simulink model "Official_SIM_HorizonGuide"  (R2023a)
settings: Solver=ode4  StartTime=0.0  StopTime=100  FixedStep=0.01  RelTol=1e-3
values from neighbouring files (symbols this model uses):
  Aeq = zeros(6*N+3*(N-1),6*N+3*(N-1))    [Input_Official_SIM.m]
  c = 1e-4    (= 0.0001)    [Input_Official_SIM.m]
  dt = 8    [Input_Official_SIM.m]
  dyn_s = 1e3    (= 1000)    [Input_Official_SIM.m]
  F_D = -1/2*rho*CD*S*Vx^2    (= -0.0398770126883)    [Input_Official_SIM.m]
  Fj2 = -m_c*((3*J2*mu*(r_E^2))/(2*(r^4)))    (= -0.00135234249549)    [Input_Official_SIM.m]
  G = c*(lambda_low-lambda_top)/(sigma_0)    (= -0.03998)    [Input_Official_SIM.m]
  K_v = 20    [Input_Official_SIM.m]
  k_x = 2    [Input_Official_SIM.m]
  k_y = 0.2    [Input_Official_SIM.m]
  k_z = 2    [Input_Official_SIM.m]
  KF = 12.5*2    (= 25)    [Input_Official_SIM.m]
  lambda_low = 0.0001    [Input_Official_SIM.m]
  lambda_top = 0.2    [Input_Official_SIM.m]
  m_c = 130    [Input_Official_SIM.m]
  m_c0 = 130    [Input_Official_SIM.m]
  N = 20    [Input_Official_SIM.m]
  omega_0 = (mu/r^3)^0.5    (= 0.00105684438429)    [Input_Official_SIM.m]
  sigma_0 = 5e-4    (= 0.0005)    [Input_Official_SIM.m]
  tau = 1    [Input_Official_SIM.m]
  U_off = 0.2    [Input_Official_SIM.m]
  U_on = 0.75    [Input_Official_SIM.m]
  Umax = 2    [Input_Official_SIM.m]
  updaterate = 2    [Input_Official_SIM.m]
  x0 = -200    [Input_Official_SIM.m]
  x0_dot = 3/2*omega_0*z0    (= 0.158526657643)    [Input_Official_SIM.m]
  y0 = 0    [Input_Official_SIM.m]
  y0_dot = 0    [Input_Official_SIM.m]
  z0 = 100    [Input_Official_SIM.m]
  z0_dot = 0    [Input_Official_SIM.m]
undefined symbols (not defined in the file or in its folder): DiscIntNeverNeededParam

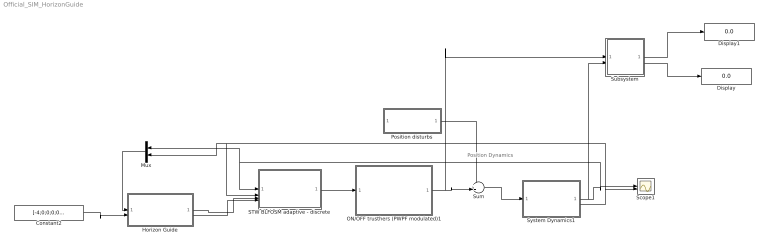
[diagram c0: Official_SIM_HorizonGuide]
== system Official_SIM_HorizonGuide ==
  note: Position Dynamics
  Constant2 : Constant  Value=[-4;0;0;0;0;0]
  Display : Display
  Display1 : Display
  Horizon Guide : Subsystem  TreatAsAtomicUnit=on
  Mux : Mux  Inputs=2
  ON/OFF trusthers (PWPF modulated)1 : Subsystem
  Position disturbs : Subsystem
  STW BLFOSM adaptive - discrete : Subsystem  TreatAsAtomicUnit=on  SystemSampleTime=0.1
  Scope1 : Scope  NumInputPorts=2
  Subsystem : Subsystem
  Sum : Sum  Inputs=++|
  System Dynamics1 : Subsystem
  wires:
  Horizon Guide/1(x_Des) -> STW BLFOSM adaptive - discrete/3(x_des)
  System Dynamics1/2(x_dot) -> STW BLFOSM adaptive - discrete/2(x_dot_live), Mux/2, Scope1/2
  Constant2/1 -> Horizon Guide/2(x_target)
  Sum/1 -> System Dynamics1/1(F)
  Mux/1 -> Horizon Guide/1(x_start)
  Horizon Guide/2(x_dot_dest) -> STW BLFOSM adaptive - discrete/4(x_dot_des)
  System Dynamics1/1(x) -> Subsystem/2(x), STW BLFOSM adaptive - discrete/1(x_live), Mux/1, Scope1/1
  Position disturbs/1(Out1) -> Sum/1
  STW BLFOSM adaptive - discrete/1(Trust) -> ON/OFF trusthers (PWPF modulated)1/1(In1)
  ON/OFF trusthers (PWPF modulated)1/1(F) -> Subsystem/1(F), Sum/2
  Subsystem/2(Endtime) -> Display/1
  Subsystem/1(Prop) -> Display1/1

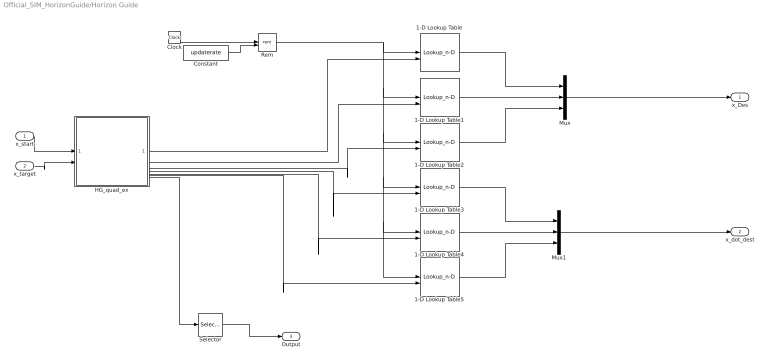
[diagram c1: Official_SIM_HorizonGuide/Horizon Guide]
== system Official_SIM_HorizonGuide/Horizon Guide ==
  x_start : Inport
  x_target : Inport  Port=2
  1-D Lookup Table{,1..5} (6 alike) : Lookup_n-D  NumberOfTableDimensions=1  BreakpointsForDimension1=[0:dt:(N-1)*dt]  TableSource=Input port  Table=tanh([-5:5])  InterpMethod=Cubic spline  InternalRulePriority=Speed  RndMeth=Simplest
  Clock : Clock
  Constant : Constant  Value=updaterate
  HG_quad_ex : MATLAB Function  TreatAsAtomicUnit=on  SystemSampleTime=updaterate
  Mux : Mux  Inputs=3
  Mux1 : Mux  Inputs=3
  Rem : Math  Operator=rem
  Selector : Selector  NumberOfDimensions=2  InputPortWidth=3  IndexOptions=Index vector (dialog),Index vector (dialog)  Indices=[1:3],1  OutputSizes=1,1
  x_Des : Outport
  x_dot_dest : Outport  Port=2
  Output : Outport  Port=3
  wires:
  Constant/1 -> Rem/2
  Rem/1 -> 1-D Lookup Table5/1, 1-D Lookup Table4/1, 1-D Lookup Table3/1, 1-D Lookup Table2/1, 1-D Lookup Table1/1, 1-D Lookup Table/1
  Clock/1 -> Rem/1
  Mux/1 -> x_Des/1
  Mux1/1 -> x_dot_dest/1
  1-D Lookup Table/1 -> Mux/1
  1-D Lookup Table1/1 -> Mux/2
  1-D Lookup Table2/1 -> Mux/3
  1-D Lookup Table3/1 -> Mux1/1
  1-D Lookup Table4/1 -> Mux1/2
  1-D Lookup Table5/1 -> Mux1/3
  HG_quad_ex/1(x) -> 1-D Lookup Table/2
  HG_quad_ex/2(y) -> 1-D Lookup Table1/2
  HG_quad_ex/3(z) -> 1-D Lookup Table2/2
  HG_quad_ex/4(x_dot) -> 1-D Lookup Table3/2
  HG_quad_ex/5(y_dot) -> 1-D Lookup Table4/2
  HG_quad_ex/6(z_dot) -> 1-D Lookup Table5/2
  HG_quad_ex/7(u) -> Selector/1
  Selector/1 -> Output/1
  x_start/1 -> HG_quad_ex/1(x_start)
  x_target/1 -> HG_quad_ex/2(x_target)

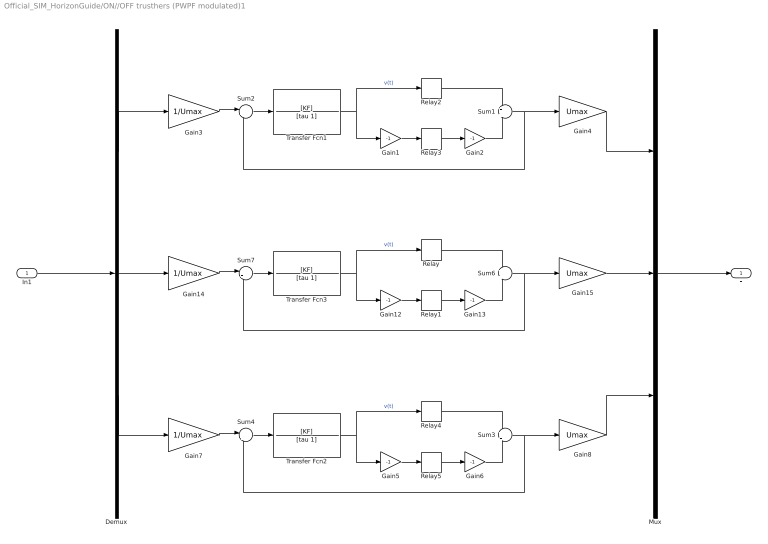
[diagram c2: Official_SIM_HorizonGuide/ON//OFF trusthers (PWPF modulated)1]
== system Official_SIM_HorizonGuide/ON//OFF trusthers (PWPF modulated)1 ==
  In1 : Inport
  Demux : Demux  Outputs=3
  Gain{1..2,5..6,12..13} (6 alike) : Gain  Gain=-1
  Gain14 : Gain  Gain=1/Umax  Multiplication=Matrix(K*u)
  Gain15 : Gain  Gain=Umax  Multiplication=Matrix(K*u)
  Gain3 : Gain  Gain=1/Umax  Multiplication=Matrix(K*u)
  Gain4 : Gain  Gain=Umax  Multiplication=Matrix(K*u)
  Gain7 : Gain  Gain=1/Umax  Multiplication=Matrix(K*u)
  Gain8 : Gain  Gain=Umax  Multiplication=Matrix(K*u)
  Mux : Mux  Inputs=3
  Relay{,1..5} (6 alike) : Relay  OnSwitchValue=U_on  OffSwitchValue=U_off
  Sum1 : Sum  Inputs=+|+
  Sum2 : Sum  Inputs=|+-
  Sum3 : Sum  Inputs=+|+
  Sum4 : Sum  Inputs=|+-
  Sum6 : Sum  Inputs=+|+
  Sum7 : Sum  Inputs=|+-
  Transfer Fcn1 : TransferFcn  Numerator=[KF]  Denominator=[tau 1]
  Transfer Fcn2 : TransferFcn  Numerator=[KF]  Denominator=[tau 1]
  Transfer Fcn3 : TransferFcn  Numerator=[KF]  Denominator=[tau 1]
  F : Outport
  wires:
  Relay/1 -> Sum6/1
  In1/1 -> Demux/1
  Relay3/1 -> Gain2/1
  Demux/3 -> Gain7/1
  Demux/2 -> Gain14/1
  Sum2/1 -> Transfer Fcn1/1
  Relay2/1 -> Sum1/1
  Sum7/1 -> Transfer Fcn3/1
  Gain6/1 -> Sum3/2
  Relay5/1 -> Gain6/1
  Gain2/1 -> Sum1/2
  Sum6/1 -> Gain15/1, Sum7/2
  Relay1/1 -> Gain13/1
  Sum3/1 -> Gain8/1, Sum4/2
  Gain7/1 -> Sum4/1
  Gain12/1 -> Relay1/1
  Transfer Fcn2/1 -> Gain5/1, Relay4/1  "v(t)"
  Gain1/1 -> Relay3/1
  Gain5/1 -> Relay5/1
  Sum1/1 -> Gain4/1, Sum2/2
  Gain13/1 -> Sum6/2
  Relay4/1 -> Sum3/1
  Sum4/1 -> Transfer Fcn2/1
  Transfer Fcn3/1 -> Gain12/1, Relay/1  "v(t)"
  Gain3/1 -> Sum2/1
  Transfer Fcn1/1 -> Gain1/1, Relay2/1  "v(t)"
  Gain14/1 -> Sum7/1
  Gain15/1 -> Mux/2
  Gain4/1 -> Mux/1
  Gain8/1 -> Mux/3
  Demux/1 -> Gain3/1
  Mux/1 -> F/1

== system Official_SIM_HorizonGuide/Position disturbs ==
  Constant : Constant  Value=F_D+Fj2
  Constant1 : Constant  Value=0
  Constant2 : Constant  Value=0
  Mux : Mux  Inputs=3
  Out1 : Outport
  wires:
  Constant/1 -> Mux/1
  Mux/1 -> Out1/1
  Constant1/1 -> Mux/2
  Constant2/1 -> Mux/3

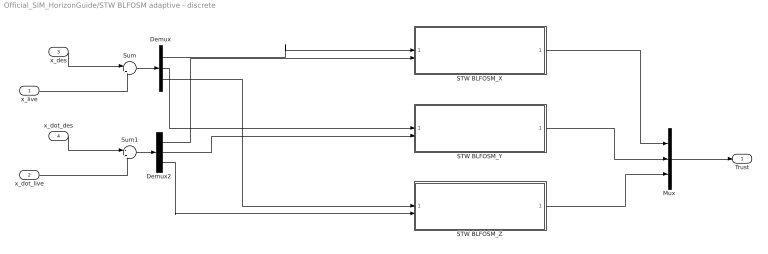
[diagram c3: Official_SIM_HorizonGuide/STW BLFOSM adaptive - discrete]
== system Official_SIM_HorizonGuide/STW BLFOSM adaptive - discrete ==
  x_live : Inport
  x_dot_live : Inport  Port=2
  x_des : Inport  Port=3
  x_dot_des : Inport  Port=4
  Demux : Demux  Outputs=3
  Demux2 : Demux  Outputs=3
  Mux : Mux  Inputs=3
  STW BLFOSM_X : Subsystem
  STW BLFOSM_Y : Subsystem
  STW BLFOSM_Z : Subsystem
  Sum : Sum  Inputs=-|+
  Sum1 : Sum  Inputs=-|+
  Trust : Outport
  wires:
  STW BLFOSM_Z/1(T_X) -> Mux/3
  STW BLFOSM_Y/1(T_X) -> Mux/2
  STW BLFOSM_X/1(T_X) -> Mux/1
  x_dot_live/1 -> Sum1/2
  x_dot_des/1 -> Sum1/1
  Sum1/1 -> Demux2/1
  Demux/3 -> STW BLFOSM_Z/1(x_e)
  Demux/2 -> STW BLFOSM_Y/1(x_e)
  Demux/1 -> STW BLFOSM_X/1(x_e)
  Sum/1 -> Demux/1
  x_des/1 -> Sum/1
  x_live/1 -> Sum/2
  Demux2/3 -> STW BLFOSM_Z/2(x_e_dot)
  Demux2/2 -> STW BLFOSM_Y/2(x_e_dot)
  Demux2/1 -> STW BLFOSM_X/2(x_e_dot)
  Mux/1 -> Trust/1

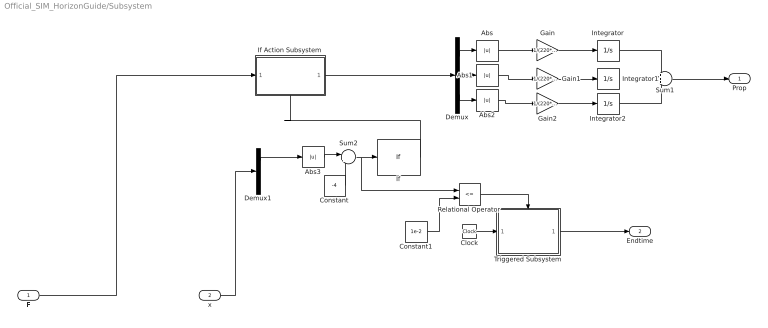
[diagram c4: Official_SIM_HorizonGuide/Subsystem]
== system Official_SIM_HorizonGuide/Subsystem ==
  F : Inport
  x : Inport  Port=2
  Abs{,1..3} (4 alike) : Abs
  Clock : Clock
  Constant : Constant  Value=-4
  Constant1 : Constant  Value=1e-2
  Demux : Demux  Outputs=3
  Demux1 : Demux  Outputs=3
  Gain : Gain  Gain=1/(220*9.81)
  Gain1 : Gain  Gain=1/(220*9.81)
  Gain2 : Gain  Gain=1/(220*9.81)
  If : If  IfExpression=u1 >= 1e-2  ShowElse=off
  If Action Subsystem : Subsystem  TreatAsAtomicUnit=on
  Integrator : Integrator
  Integrator1 : Integrator
  Integrator2 : Integrator
  Relational Operator : RelationalOperator  Operator=<=  OutDataTypeStr=boolean  RndMeth=Simplest
  Sum1 : Sum  Inputs=+++
  Sum2 : Sum  Inputs=|++
  Triggered Subsystem : Subsystem  TreatAsAtomicUnit=on
  Prop : Outport
  Endtime : Outport  Port=2
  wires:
  Gain2/1 -> Integrator2/1
  Demux/1 -> Abs/1
  Abs1/1 -> Gain1/1
  Abs2/1 -> Gain2/1
  Demux1/1 -> Abs3/1
  Gain/1 -> Integrator/1
  Gain1/1 -> Integrator1/1
  Integrator/1 -> Sum1/1
  Demux/3 -> Abs2/1
  Sum1/1 -> Prop/1
  Integrator2/1 -> Sum1/3
  Constant/1 -> Sum2/2
  F/1 -> If Action Subsystem/1(F)
  Abs/1 -> Gain/1
  Demux/2 -> Abs1/1
  Sum2/1 -> Relational Operator/1, If/1
  If/1 -> If Action Subsystem/Action
  Abs3/1 -> Sum2/1
  If Action Subsystem/1(Out1) -> Demux/1
  Integrator1/1 -> ?
  x/1 -> Demux1/1
  Triggered Subsystem/1(Out1) -> Endtime/1
  Relational Operator/1 -> Triggered Subsystem/Trigger
  Constant1/1 -> Relational Operator/2
  Clock/1 -> Triggered Subsystem/1(Input)

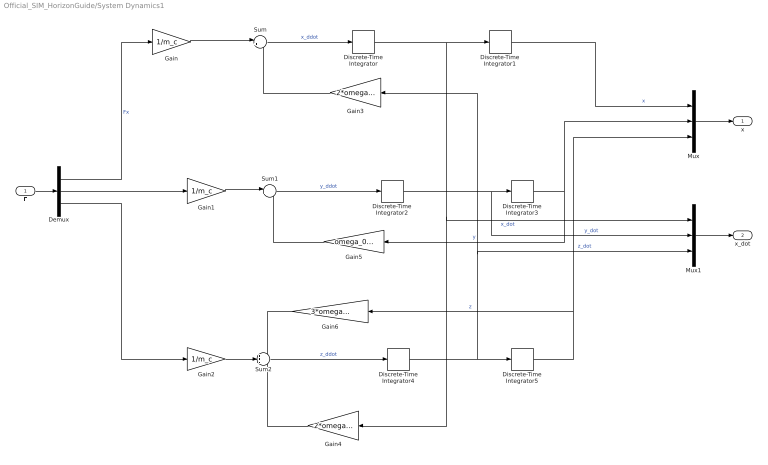
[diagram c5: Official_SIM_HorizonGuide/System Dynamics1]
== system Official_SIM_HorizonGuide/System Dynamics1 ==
  F : Inport
  Demux : Demux  Outputs=3
  Discrete-Time Integrator : DiscreteIntegrator  InitialCondition=x0_dot  SampleTime=-1  ICPrevOutput=DiscIntNeverNeededParam  ICPrevScaledInput=DiscIntNeverNeededParam
  Discrete-Time Integrator1 : DiscreteIntegrator  InitialCondition=x0  SampleTime=-1  ICPrevOutput=DiscIntNeverNeededParam  ICPrevScaledInput=DiscIntNeverNeededParam
  Discrete-Time Integrator2 : DiscreteIntegrator  InitialCondition=y0_dot  SampleTime=-1  ICPrevOutput=DiscIntNeverNeededParam  ICPrevScaledInput=DiscIntNeverNeededParam
  Discrete-Time Integrator3 : DiscreteIntegrator  InitialCondition=y0  SampleTime=-1  ICPrevOutput=DiscIntNeverNeededParam  ICPrevScaledInput=DiscIntNeverNeededParam
  Discrete-Time Integrator4 : DiscreteIntegrator  InitialCondition=z0_dot  SampleTime=-1  ICPrevOutput=DiscIntNeverNeededParam  ICPrevScaledInput=DiscIntNeverNeededParam
  Discrete-Time Integrator5 : DiscreteIntegrator  InitialCondition=z0  SampleTime=-1  ICPrevOutput=DiscIntNeverNeededParam  ICPrevScaledInput=DiscIntNeverNeededParam
  Gain : Gain  Gain=1/m_c
  Gain1 : Gain  Gain=1/m_c
  Gain2 : Gain  Gain=1/m_c
  Gain3 : Gain  Gain=2*omega_0
  Gain4 : Gain  Gain=2*omega_0
  Gain5 : Gain  Gain=omega_0^2
  Gain6 : Gain  Gain=3*omega_0^2
  Mux : Mux  Inputs=3
  Mux1 : Mux  Inputs=3
  Sum : Sum  Inputs=|++
  Sum1 : Sum  Inputs=|+-
  Sum2 : Sum  Inputs=++-
  x : Outport  PortDimensions=3
  x_dot : Outport  Port=2
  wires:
  F/1 -> Demux/1
  Demux/1 -> Gain/1  "Fx"
  Demux/2 -> Gain1/1
  Demux/3 -> Gain2/1
  Discrete-Time Integrator/1 -> Discrete-Time Integrator1/1, Mux1/1, Gain4/1  "x_dot"
  Gain/1 -> Sum/1
  Gain3/1 -> Sum/2
  Sum/1 -> Discrete-Time Integrator/1  "x_ddot"
  Discrete-Time Integrator3/1 -> Mux/2, Gain5/1  "y"
  Discrete-Time Integrator2/1 -> Discrete-Time Integrator3/1, Mux1/2  "y_dot"
  Sum1/1 -> Discrete-Time Integrator2/1  "y_ddot"
  Discrete-Time Integrator4/1 -> Discrete-Time Integrator5/1, Mux1/3, Gain3/1  "z_dot"
  Discrete-Time Integrator5/1 -> Mux/3, Gain6/1  "z"
  Sum2/1 -> Discrete-Time Integrator4/1  "z_ddot"
  Gain5/1 -> Sum1/2
  Gain1/1 -> Sum1/1
  Gain4/1 -> Sum2/3
  Gain6/1 -> Sum2/1
  Gain2/1 -> Sum2/2
  Mux/1 -> x/1
  Mux1/1 -> x_dot/1
  Discrete-Time Integrator1/1 -> Mux/1  "x"

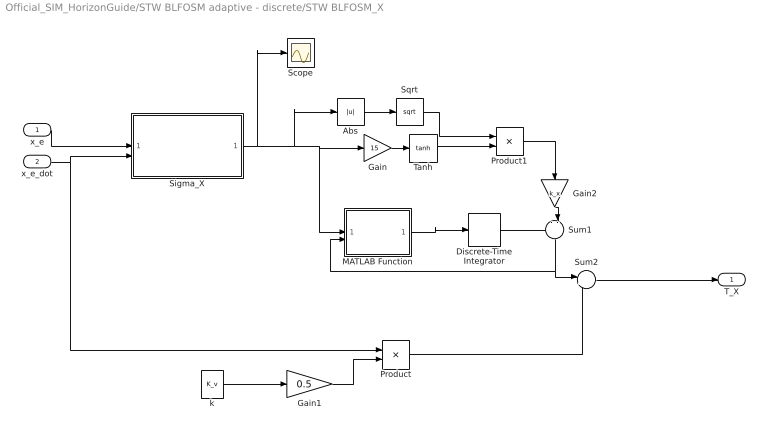
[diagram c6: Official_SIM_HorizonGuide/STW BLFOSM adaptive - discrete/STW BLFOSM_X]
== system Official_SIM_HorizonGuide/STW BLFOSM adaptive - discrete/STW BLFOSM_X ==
  x_e : Inport
  x_e_dot : Inport  Port=2
  Abs : Abs
  Discrete-Time Integrator : DiscreteIntegrator  SampleTime=-1  ICPrevOutput=DiscIntNeverNeededParam  ICPrevScaledInput=DiscIntNeverNeededParam
  Gain : Gain  Gain=15
  Gain1 : Gain  Gain=0.5
  Gain2 : Gain  Gain=k_x
  MATLAB Function : MATLAB Function  TreatAsAtomicUnit=on
  Product : Product
  Product1 : Product
  Scope : Scope
  Sigma_X : Subsystem
  Sqrt : Sqrt
  Sum1 : Sum  Inputs=--|
  Sum2 : Sum  Inputs=|+-
  Tanh : Trigonometry  Operator=tanh
  k : Constant  Value=K_v
  T_X : Outport
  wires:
  Sqrt/1 -> Product1/1
  Sum1/1 -> Sum2/1, MATLAB Function/2(u)
  x_e_dot/1 -> Sigma_X/2(x_dot_live), Product/1
  Product/1 -> Sum2/2
  Gain1/1 -> Product/2
  k/1 -> Gain1/1
  x_e/1 -> Sigma_X/1(x_e)
  Product1/1 -> Gain2/1
  Sigma_X/1(Sigma_X) -> Scope/1, Gain/1, MATLAB Function/1(sigma), Abs/1
  Gain2/1 -> Sum1/2
  Discrete-Time Integrator/1 -> Sum1/1
  MATLAB Function/1(u1) -> Discrete-Time Integrator/1
  Abs/1 -> Sqrt/1
  Sum2/1 -> T_X/1
  Tanh/1 -> Product1/2
  Gain/1 -> Tanh/1

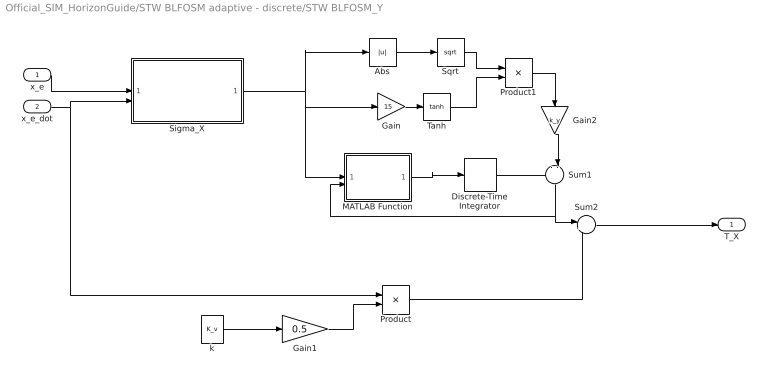
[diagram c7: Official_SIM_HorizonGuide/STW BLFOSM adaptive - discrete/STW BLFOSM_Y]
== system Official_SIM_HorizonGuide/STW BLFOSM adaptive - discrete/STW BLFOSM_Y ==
  x_e : Inport
  x_e_dot : Inport  Port=2
  Abs : Abs
  Discrete-Time Integrator : DiscreteIntegrator  SampleTime=-1  ICPrevOutput=DiscIntNeverNeededParam  ICPrevScaledInput=DiscIntNeverNeededParam
  Gain : Gain  Gain=15
  Gain1 : Gain  Gain=0.5
  Gain2 : Gain  Gain=k_y
  MATLAB Function : MATLAB Function  TreatAsAtomicUnit=on
  Product : Product
  Product1 : Product
  Sigma_X : Subsystem
  Sqrt : Sqrt
  Sum1 : Sum  Inputs=--|
  Sum2 : Sum  Inputs=|+-
  Tanh : Trigonometry  Operator=tanh
  k : Constant  Value=K_v
  T_X : Outport
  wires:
  Sum2/1 -> T_X/1
  MATLAB Function/1(u1) -> Discrete-Time Integrator/1
  Discrete-Time Integrator/1 -> Sum1/1
  Gain2/1 -> Sum1/2
  x_e/1 -> Sigma_X/1(x_e)
  k/1 -> Gain1/1
  Gain1/1 -> Product/2
  Product/1 -> Sum2/2
  x_e_dot/1 -> Product/1, Sigma_X/2(x_dot_live)
  Sum1/1 -> MATLAB Function/2(u), Sum2/1
  Abs/1 -> Sqrt/1
  Tanh/1 -> Product1/2
  Sigma_X/1(Sigma_X) -> Gain/1, MATLAB Function/1(sigma), Abs/1
  Sqrt/1 -> Product1/1
  Product1/1 -> Gain2/1
  Gain/1 -> Tanh/1

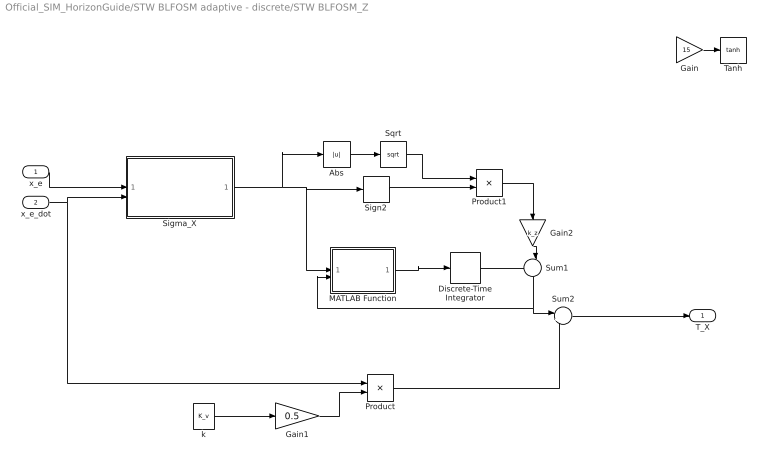
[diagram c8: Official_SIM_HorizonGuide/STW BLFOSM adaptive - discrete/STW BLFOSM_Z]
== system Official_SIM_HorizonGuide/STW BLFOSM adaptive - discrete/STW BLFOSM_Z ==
  x_e : Inport
  x_e_dot : Inport  Port=2
  Abs : Abs
  Discrete-Time Integrator : DiscreteIntegrator  SampleTime=-1  ICPrevOutput=DiscIntNeverNeededParam  ICPrevScaledInput=DiscIntNeverNeededParam
  Gain : Gain  Commented=on  Gain=15
  Gain1 : Gain  Gain=0.5
  Gain2 : Gain  Gain=k_z
  MATLAB Function : MATLAB Function  TreatAsAtomicUnit=on
  Product : Product
  Product1 : Product
  Sigma_X : Subsystem
  Sign2 : Signum
  Sqrt : Sqrt
  Sum1 : Sum  Inputs=--|
  Sum2 : Sum  Inputs=|+-
  Tanh : Trigonometry  Commented=on  Operator=tanh
  k : Constant  Value=K_v
  T_X : Outport
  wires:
  Sqrt/1 -> Product1/1
  Sum1/1 -> Sum2/1, MATLAB Function/2(u)
  x_e_dot/1 -> Sigma_X/2(x_dot_live), Product/1
  Product/1 -> Sum2/2
  Gain1/1 -> Product/2
  k/1 -> Gain1/1
  x_e/1 -> Sigma_X/1(x_e)
  Product1/1 -> Gain2/1
  Sigma_X/1(Sigma_X) -> Sign2/1, MATLAB Function/1(sigma), Abs/1
  Gain2/1 -> Sum1/2
  Discrete-Time Integrator/1 -> Sum1/1
  MATLAB Function/1(u1) -> Discrete-Time Integrator/1
  Abs/1 -> Sqrt/1
  Sum2/1 -> T_X/1
  Sign2/1 -> Product1/2
  Gain/1 -> Tanh/1

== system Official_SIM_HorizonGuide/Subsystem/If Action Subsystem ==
  F : Inport
  Action Port : ActionPort  ActionPortLabel=if(u1 >= 1e-2)
  Out1 : Outport
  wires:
  F/1 -> Out1/1

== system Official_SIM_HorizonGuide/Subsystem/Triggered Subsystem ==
  Input : Inport
  Trigger : TriggerPort  VariantControl=(inherit)
  Out1 : Outport
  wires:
  Input/1 -> Out1/1

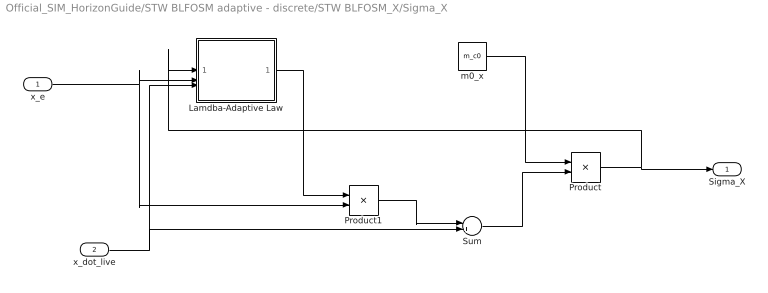
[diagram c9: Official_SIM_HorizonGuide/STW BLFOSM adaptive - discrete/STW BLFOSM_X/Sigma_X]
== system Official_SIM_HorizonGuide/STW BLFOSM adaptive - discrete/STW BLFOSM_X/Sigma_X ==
  x_e : Inport
  x_dot_live : Inport  Port=2
  Lamdba-Adaptive Law : Subsystem
  Product : Product
  Product1 : Product
  Sum : Sum  Inputs=|++
  m0_x : Constant  Value=m_c0
  Sigma_X : Outport
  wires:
  x_dot_live/1 -> Lamdba-Adaptive Law/3(x_dot_live), Sum/2
  Product/1 -> Lamdba-Adaptive Law/1(Sigma), Sigma_X/1
  m0_x/1 -> Product/1
  Sum/1 -> Product/2
  Product1/1 -> Sum/1
  Lamdba-Adaptive Law/1(Lambda) -> Product1/1
  x_e/1 -> Product1/2, Lamdba-Adaptive Law/2(x_err)

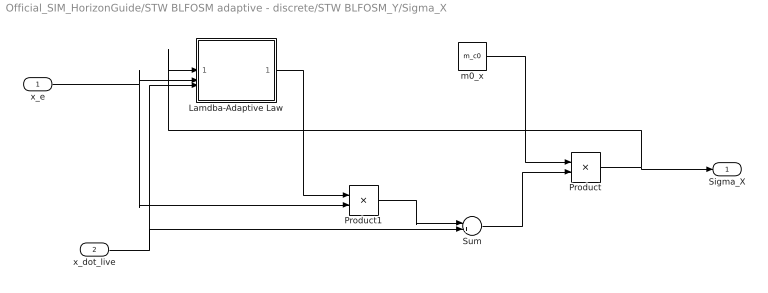
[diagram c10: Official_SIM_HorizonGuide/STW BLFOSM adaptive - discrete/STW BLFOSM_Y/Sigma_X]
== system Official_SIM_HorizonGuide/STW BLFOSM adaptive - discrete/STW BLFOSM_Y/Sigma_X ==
  x_e : Inport
  x_dot_live : Inport  Port=2
  Lamdba-Adaptive Law : Subsystem
  Product : Product
  Product1 : Product
  Sum : Sum  Inputs=|++
  m0_x : Constant  Value=m_c0
  Sigma_X : Outport
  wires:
  x_e/1 -> Lamdba-Adaptive Law/2(x_err), Product1/2
  Lamdba-Adaptive Law/1(Lambda) -> Product1/1
  Product1/1 -> Sum/1
  Sum/1 -> Product/2
  m0_x/1 -> Product/1
  Product/1 -> Sigma_X/1, Lamdba-Adaptive Law/1(Sigma)
  x_dot_live/1 -> Sum/2, Lamdba-Adaptive Law/3(x_dot_live)

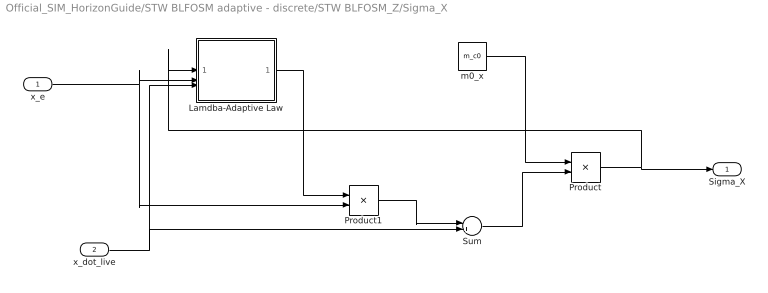
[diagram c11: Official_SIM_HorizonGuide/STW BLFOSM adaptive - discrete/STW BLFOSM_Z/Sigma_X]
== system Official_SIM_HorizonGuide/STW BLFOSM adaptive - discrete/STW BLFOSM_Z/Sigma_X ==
  x_e : Inport
  x_dot_live : Inport  Port=2
  Lamdba-Adaptive Law : Subsystem
  Product : Product
  Product1 : Product
  Sum : Sum  Inputs=|++
  m0_x : Constant  Value=m_c0
  Sigma_X : Outport
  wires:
  x_dot_live/1 -> Lamdba-Adaptive Law/3(x_dot_live), Sum/2
  Product/1 -> Lamdba-Adaptive Law/1(Sigma), Sigma_X/1
  m0_x/1 -> Product/1
  Sum/1 -> Product/2
  Product1/1 -> Sum/1
  Lamdba-Adaptive Law/1(Lambda) -> Product1/1
  x_e/1 -> Product1/2, Lamdba-Adaptive Law/2(x_err)

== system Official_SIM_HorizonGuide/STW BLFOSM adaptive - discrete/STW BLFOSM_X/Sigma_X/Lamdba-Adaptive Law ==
  Sigma : Inport
  x_err : Inport  Port=2
  x_dot_live : Inport  Port=3
  Discrete-Time Integrator : DiscreteIntegrator  InitialCondition=lambda_low  SampleTime=-1  ICPrevOutput=DiscIntNeverNeededParam  ICPrevScaledInput=DiscIntNeverNeededParam
  MATLAB Function : MATLAB Function  TreatAsAtomicUnit=on
  Lambda : Outport
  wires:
  MATLAB Function/1(lambda_dot) -> Discrete-Time Integrator/1
  x_err/1 -> MATLAB Function/1(x_e)
  Sigma/1 -> MATLAB Function/4(sigma)
  Discrete-Time Integrator/1 -> MATLAB Function/3(lambda), Lambda/1
  x_dot_live/1 -> MATLAB Function/2(x_e_dot)

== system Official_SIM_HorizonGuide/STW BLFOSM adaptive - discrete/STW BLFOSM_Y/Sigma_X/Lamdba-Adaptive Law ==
  Sigma : Inport
  x_err : Inport  Port=2
  x_dot_live : Inport  Port=3
  Discrete-Time Integrator : DiscreteIntegrator  InitialCondition=lambda_low  SampleTime=-1  ICPrevOutput=DiscIntNeverNeededParam  ICPrevScaledInput=DiscIntNeverNeededParam
  MATLAB Function : MATLAB Function  TreatAsAtomicUnit=on
  Lambda : Outport
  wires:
  x_dot_live/1 -> MATLAB Function/2(x_e_dot)
  Discrete-Time Integrator/1 -> Lambda/1, MATLAB Function/3(lambda)
  Sigma/1 -> MATLAB Function/4(sigma)
  x_err/1 -> MATLAB Function/1(x_e)
  MATLAB Function/1(lambda_dot) -> Discrete-Time Integrator/1

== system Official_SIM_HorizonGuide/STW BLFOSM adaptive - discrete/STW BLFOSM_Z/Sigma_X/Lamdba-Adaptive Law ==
  Sigma : Inport
  x_err : Inport  Port=2
  x_dot_live : Inport  Port=3
  Discrete-Time Integrator : DiscreteIntegrator  InitialCondition=lambda_low  SampleTime=-1  ICPrevOutput=DiscIntNeverNeededParam  ICPrevScaledInput=DiscIntNeverNeededParam
  MATLAB Function : MATLAB Function  TreatAsAtomicUnit=on
  Lambda : Outport
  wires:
  MATLAB Function/1(lambda_dot) -> Discrete-Time Integrator/1
  x_err/1 -> MATLAB Function/1(x_e)
  Sigma/1 -> MATLAB Function/4(sigma)
  Discrete-Time Integrator/1 -> MATLAB Function/3(lambda), Lambda/1
  x_dot_live/1 -> MATLAB Function/2(x_e_dot)

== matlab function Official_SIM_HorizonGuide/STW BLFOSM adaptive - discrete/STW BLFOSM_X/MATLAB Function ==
function u1 = fcn(sigma, u, alpha_x)
u1 = 0;
if abs(u) < 2
    % u1 = alpha_x*sign(sigma);
    u1 = alpha_x*tanh(15*sigma);
else
    u1 = u;
end

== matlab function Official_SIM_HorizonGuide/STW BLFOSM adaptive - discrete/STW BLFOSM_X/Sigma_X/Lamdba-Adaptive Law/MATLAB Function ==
function lambda_dot = fcn(x_e,x_e_dot, lambda,sigma, sigma_0, lambda_top,c, G, lambda_low)
eta = sigma;
lambda_dot = lambda_low;
if sigma > sigma_0
    eta = sigma;
else 
    eta = 0;
h = G*eta*sign(x_e)-c*(lambda-lambda_top);
if lambda == lambda_low 
    lambda_dot = max(0,h);
end
if lambda < lambda_top && lambda > lambda_low
    lambda_dot = h;
end
if lambda == lambda_top
    lambda_dot = min(0,h);
end

end

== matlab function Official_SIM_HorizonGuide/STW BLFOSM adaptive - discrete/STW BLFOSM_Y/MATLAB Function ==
function u1 = fcn(sigma, u, alpha_y)
u1 = 0;
if abs(u) < 2
    u1 = alpha_y*sign(sigma);
else
    u1 = u;
end

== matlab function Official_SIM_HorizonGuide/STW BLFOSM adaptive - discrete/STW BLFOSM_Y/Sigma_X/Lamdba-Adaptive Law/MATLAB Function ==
function lambda_dot = fcn(x_e,x_e_dot, lambda,sigma, sigma_0, lambda_top,c, G, lambda_low)
eta = sigma;
lambda_dot = lambda_low;
if sigma > sigma_0
    eta = sigma;
else 
    eta = 0;
h = G*eta*sign(x_e)-c*(lambda-lambda_top);
if lambda == lambda_low 
    lambda_dot = max(0,h);
end
if lambda < lambda_top && lambda > lambda_low
    lambda_dot = h;
end
if lambda == lambda_top
    lambda_dot = min(0,h);
end

end

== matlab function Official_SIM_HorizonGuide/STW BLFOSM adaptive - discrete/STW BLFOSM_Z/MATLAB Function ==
function u1 = fcn(sigma, u, alpha_z)
u1 = 0;
if abs(u) < 2
    u1 = alpha_z*sign(sigma);
    % u1 = alpha_z*tanh(15*sigma);
else
    u1 = u;
end

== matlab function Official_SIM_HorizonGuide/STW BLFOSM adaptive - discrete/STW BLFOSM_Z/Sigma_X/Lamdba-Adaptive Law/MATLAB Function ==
function lambda_dot = fcn(x_e,x_e_dot, lambda,sigma, sigma_0, lambda_top,c, G, lambda_low)
eta = sigma;
lambda_dot = lambda_low;
if sigma > sigma_0
    eta = sigma;
else 
    eta = 0;
h = G*eta*sign(x_e)-c*(lambda-lambda_top);
if lambda == lambda_low 
    lambda_dot = max(0,h);
end
if lambda < lambda_top && lambda > lambda_low
    lambda_dot = h;
end
if lambda == lambda_top
    lambda_dot = min(0,h);
end

end

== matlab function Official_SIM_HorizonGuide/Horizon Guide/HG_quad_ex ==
function [x,y,z,x_dot,y_dot,z_dot,u] = HorizonGuide(N,dt,dyn_s,Aeq, x_start, x_target)

max_vel = 0.5;
beq =[x_start-x_target;zeros(size(Aeq,2)-6,1)]/dyn_s;

Aeq = [Aeq;-Aeq];
beq = [beq;-beq];

beq_out = [x_start+[500 0 0 0 0 0]';zeros( size(Aeq,2)-6,1)]/dyn_s;

beq_out = [beq_out;-beq_out];

%%Control bounds
Acontrolup = [zeros(3*(N-1),6*N), diag(ones(3*(N-1),1))];
bcontrolup = 2*ones((N-1)*3,1);
Acontroldown  =  [zeros(3*(N-1),6*N), -diag(ones(3*(N-1),1))];
bcontroldown = 2*ones((N-1)*3,1);
Acontrol = [Acontrolup;Acontroldown];
bcontrol = [bcontrolup;bcontroldown]/dyn_s;

%%speed bounds Acontrolup = [zeros(3*(N-1),6*N), diag(ones(3*(N-1),1))];
Aspeedup = [diag(repmat([0 0 0 1 1 1]',N,1))  zeros(6*N,3*(N-1))];
bspeedup = max_vel*ones(6*N,1);
Aspeedlow  = [-diag(repmat([0 0 0 1 1 1]',N,1)), zeros(6*N,3*(N-1))];
bspeedlow = max_vel*ones(6*N,1);
Aspeed = [Aspeedup;Aspeedlow];
bspeed = [bspeedup;bspeedlow]/dyn_s;

%%final horizon
A_finiteup = [zeros(6,N*9-3)];
A_finitelow = [zeros(6,N*9-3)];
A_finiteup(:,6*N-5:6*N) = eye(6,6);
A_finitelow(:,6*N-5:6*N) = -eye(6,6);
b_finiteup = zeros(6,1);
b_finitelow = -zeros(6,1);


%%%%%% COST FUNCTION & CONSTRAINTS %%%%%%%%

f = zeros(9*N-3,1);
%%inside cone objective
H = diag([ 1*repmat([0 0 1e3 1e2 1e2 1e1]',N-1,1); [1 1e1 1e3 1e3 1e2 1e1]'; 1*ones(3*(N-1),1)]);
A_in = [Aeq;Acontrol;Aspeed];
b_in = [beq;bcontrol;bspeed];


%%outside cone objective 
H_out = diag([ 1*repmat([0 0 1e1 1 5e3 1e4]',N-1,1); [0 5e1 1e1 1 5e3 1e4]';1e2*ones(3*(N-1),1)]);
A_out = [Aeq;Acontrol];
b_out = [beq;bcontrol];


%%%far-range objective (Homann)
H_far_altitude = diag([1*repmat([1e-1 0 5e1 1e4 0 5e5]',N-1,1); [1 0 1e2 1e4 0 1e6]'; 1e4*ones(3*(N-1),1)]);

H_far_altitude_off = diag([1*repmat([1e-1 0 1e1 1e4 0 1e6]',N-1,1); [1 0 1e3 1e4 0 1e6]'; 1e3*ones(3*(N-1),1)]);

A_outside = [Aeq;Acontrol];
b_outside = [beq_out;bcontrol];

%%%far-range objective (Radial)
H_far_distance = diag([ 1*repmat([0 1 1e3 1e3 1e3 7.5e2]',N-1,1); [1 1e1 1e3 2e3 1e3 1e3]';1e3*ones(3*(N-1),1)]);

A_f = [A_finiteup;A_finitelow];
b_f = [b_finiteup;b_finitelow];

A_finite = [Aeq;Acontrol;Aspeed;A_f];
b_finite = [beq;bcontrol;bspeed;b_f];


%%%%%%%%%%%%%%%%% RESOLUTION %%%%%%%%
sol = zeros(6,N);
zsol = zeros(N*9-3,1);

flag=0;

if norm(x_start(1:3)-x_target(1:3)) <= 1e-1
    sol = zeros(6,N)+x_target;
    flag = 1;
end 

if norm(x_start(1:3)-x_target(1:3))/norm(x_start(4:6)) <= dt*(N-1.5) && not(flag)
    [zsol] = quad_wright(H,f,A_finite,b_finite,1000,1e-6,0);
    sol=reshape(zsol(1:N*6),6,N)*dyn_s + x_target;
    flag=1;
end

if not(flag)
    if norm(x_start(1)) <= 505 && norm(x_start(1:3))*cosd(0.1) <= norm(x_start(1))
        [zsol] = quad_wright(H,f,A_in,b_in,1000,1e-6,0);
        sol = reshape(zsol(1:N*6),6,N)*dyn_s + x_target;
    elseif norm(x_start(1)) <= 500 && norm(x_start(1:3))*cosd(0.1) >= norm(x_start(1))
        [zsol] = quad_wright(H_out,f,A_out,b_out,1000,1e-6,0);
        sol = reshape(zsol(1:N*6),6,N)*dyn_s + x_target;
       
     elseif norm(x_start(1)) >= 500 && norm(x_start(2:3)) >= 10 && x_start(3,1)>0
         [zsol] = quad_wright(H_far_altitude,f,A_outside,b_outside,1000,1e-6,0);
         sol = reshape(zsol(1:N*6),6,N)*dyn_s -[500 0 0 0 0 0]';
         
    elseif norm(x_start(1)) >= 500 && norm(x_start(2:3)) >= 10 && x_start(3,1) < 0
        [zsol] = quad_wright(H_far_altitude_off,f,A_outside,b_outside,1000,1e-6,0);
           sol = reshape(zsol(1:N*6),6,N)*dyn_s -[500 0 0 0 0 0]';
          
    elseif norm(x_start(1)) >= 500 && norm(x_start(2:3)) <= 25 
        [zsol] = quad_wright(H_far_distance,f,A_outside,b_outside,1000,1e-6,0);
        sol = reshape(zsol(1:N*6),6,N)*dyn_s -[500 0 0 0 0 0]';    
    end
end

traj = zeros(6,N);
traj(1:6,1:N) = sol;

x=     zeros(1,N);
y=     zeros(1,N);
z=     zeros(1,N);
x_dot= zeros(1,N);
y_dot= zeros(1,N);
z_dot= zeros(1,N);

x(1,1:N)=     traj(1,1:N);
y(1,1:N)=     traj(2,1:N);
z(1,1:N)=     traj(3,1:N);
x_dot(1,1:N)= traj(4,1:N);
y_dot(1,1:N)= traj(5,1:N);
z_dot(1,1:N)= traj(6,1:N);

u = reshape(zsol(N*6+1:end),N-1,3)*dyn_s;
end


function [z,exitflag] = quad_wright(H, f, A, b, maxiter, tol, verbose)%,z0,lam0,t0)
% Solve quadratic programming problem using Wright’s (1997) Method
% Minimize 1/2 * x' * H * x + f' * x
% Subject to: Ax <= b
% Copyright (C) 2009-2013 Jonathan Currie (www.i2c2.aut.ac.nz)

% Length of constraint matrix
mc = length(b);
% Number of decision variables
ndec = length(f);

% Default Args
% if nargin < 10
%     t = [];
% else
%     t = t0;
% end
% 
% if nargin < 9
%     lam = [];
% else
%     lam = lam0;
% end
% 
% if nargin < 8
%     z = [];
% else
%     z = z0;
% end

if nargin < 7 || isempty(verbose)
    verbose = 0;
end
% 
% if nargin < 6 || isempty(tol)
%     tol = 1e-6;
% end
% 
% if nargin < 5 || isempty(maxiter)
%     maxiter = 200;
% end

% Test for Warm Start
pmax = max(max(abs([H f; A b])));

if pmax > 1
    WARMVAL = sqrt(pmax);
else
    WARMVAL = 0.5;
end

% if isempty(z)
    % Cold start
    z = zeros(ndec, 1);
    lam = WARMVAL * ones(mc, 1);
    t = WARMVAL * ones(mc, 1);
    wmode = 0;
% elseif isepty(lam)
%     % Just primal
%     lam = WARMVAL * ones(mc, 1);
%     t = WARMVAL * ones(mc, 1);
%     wmode = 1;
% elseif isempty(t)
%     % Primal + dual
%     t = WARMVAL * ones(mc, 1);
%     wmode = 2;
% else
%     % All
%     wmode = 3;
% end

% Default Values
sigma = 0.1;
ascale = 1;
inftol = tol * 10;
exitflag = 1;
cholfail = 0;
mu = t' * lam / mc;
At = A';

mr2_1 = 100;
mr2 = 10;

% Initial Residuals
r1 = -H * z - At * lam - f;
r2 = -A * z + b;

% Linsolve options
opU.UT = true;
opUT.UT = true;
opUT.TRANSA = true;


% Begin Searching
for iter = 1:maxiter
    % Create common matrices
    ilam = 1./lam;
    ilamt = ilam .* t;
    lamt = lam ./ t;
    mesil = mu * sigma .* ilam;
    IGA = bsxfun(@times, A, lamt);
    
    % matrix * diagonal matrix
    igr2 = lamt .* (r2 - mesil);
    
    % Solve
    [R, p] = chol(H + At * IGA);
    if ~p
        % Exploit matrix properties for solving
        del_z = linsolve(R, linsolve(R, (r1 + At * igr2), opUT), opU);
    else
        % Not Positive Definite
        if verbose
            fprintf(2, ' (Cholesky Failed)\n');
        end
        del_z = (H + At * IGA) \ (r1 + At * igr2);
        cholfail = cholfail + 1;
        if cholfail > 2
            exitflag = -2;
            break;
        end
    % Pull back maximum step size
    ascale = ascale - 0.1;
    end
    
    del_lam = -igr2 + IGA * del_z;
    del_t = -t + mesil - ilamt .* del_lam;
    
    % Decide on a suitable affine step-length
    duals = [lam; t];
    delta = [del_lam; del_t];
    index = delta < 0;
    if any(index)
        % Solves for min ratio (max value of alpha allowed)
        alpha = 0.9995 * min(-duals(index) ./ delta(index));
    else
        alpha = 0.999995;
    end
    
    % Check for numerical problems (alpha will go negative)
    if alpha < eps(1)
        exitflag = -3;
        break;
    end
    
    % Local Scaling
    alpha = alpha * ascale;
    
    % Increment
    lam = lam + alpha * del_lam;
    t = t + alpha * del_t;
    z = z + alpha * del_z;
    
    % Update residuals
    r1 = (1 - alpha) * r1;  % equiv to r1 = -H * z - At * lam - f
    r2 = -A * z + b;
    
    % Complementarity Gap
    muold = mu;
    mu = t' * lam / mc;
    %Infeasibility Gap
    mr2_2 = mr2_1;
    mr2_1 = mr2;
    mr1 = max(abs(r1));
    mr2 = max(abs(r2 - t));
    
    phi = (max([mr1, mr2]) + t' * lam) / pmax;

% Check for NaNs
if isnan(mu) || isnan(phi)
    exitflag = -3;
    break;
end

% Check Convergence
if mu <= tol && phi <= tol
    exitflag = 1;
    return
end

% Check For Primal Infeasibility
if iter > 6 && mr2 / pmax > tol / 10
    if abs(mr2 - mr2_1) / mr2 < inftol && abs(mr2_1 - mr2_2) / mr2_1 < inftol
        if verbose
            fprintf(2, ' (Primal Infeasibility Detected)\n');
        end
        exitflag = -4;
        return;
    end
end

% Solve centering parameter (Mehrotra’s Heuristic)
sigma = min((mu / muold)^3, 0.99999);
end

% If here, either bailed on Cholesky or Iterations Expired
if exitflag == 1
    exitflag = -1;  % expired iters
end

end
